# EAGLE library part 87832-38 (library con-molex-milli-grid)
HEADER
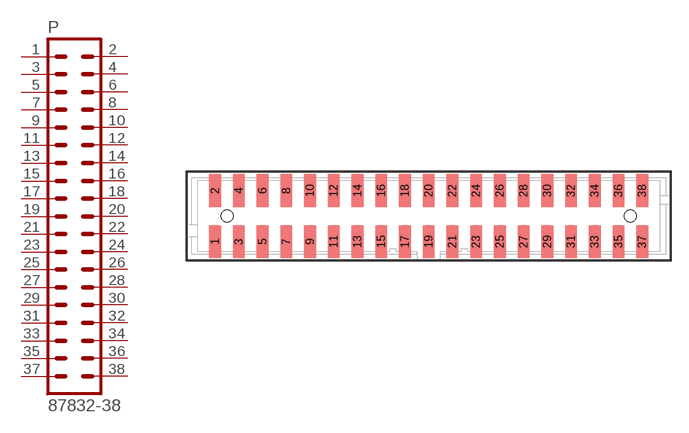
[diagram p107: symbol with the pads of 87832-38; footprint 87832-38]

Designator prefix P

## 87832-38  [87832-38]
1  1  pas
2  2  pas
3  3  pas
4  4  pas
5  5  pas
6  6  pas
7  7  pas
8  8  pas
9  9  pas
10  10  pas
11  11  pas
12  12  pas
13  13  pas
14  14  pas
15  15  pas
16  16  pas
17  17  pas
18  18  pas
19  19  pas
20  20  pas
21  21  pas
22  22  pas
23  23  pas
24  24  pas
25  25  pas
26  26  pas
27  27  pas
28  28  pas
29  29  pas
30  30  pas
31  31  pas
32  32  pas
33  33  pas
34  34  pas
35  35  pas
36  36  pas
37  37  pas
38  38  pas

## Footprint 87832-38 (pad centres in mm)
HEADER SMD Dual Row, Shrouded, Vertical
smd 1 x 2.75: 1 -18,-2.15; 2 -18,2.15; 3 -16,-2.15; 4 -16,2.15; 5 -14,-2.15; 6 -14,2.15; 7 -12,-2.15; 8 -12,2.15; 9 -10,-2.15; 10 -10,2.15; 11 -8,-2.15; 12 -8,2.15; 13 -6,-2.15; 14 -6,2.15; 15 -4,-2.15; 16 -4,2.15; 17 -2,-2.15; 18 -2,2.15; 19 0,-2.15; 20 0,2.15; 21 2,-2.15; 22 2,2.15; 23 4,-2.15; 24 4,2.15; 25 6,-2.15; 26 6,2.15; 27 8,-2.15; 28 8,2.15; 29 10,-2.15; 30 10,2.15; 31 12,-2.15; 32 12,2.15; 33 14,-2.15; 34 14,2.15; 35 16,-2.15; 36 16,2.15; 37 18,-2.15; 38 18,2.15
hole 1 at -17,0
hole 1 at 17,0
